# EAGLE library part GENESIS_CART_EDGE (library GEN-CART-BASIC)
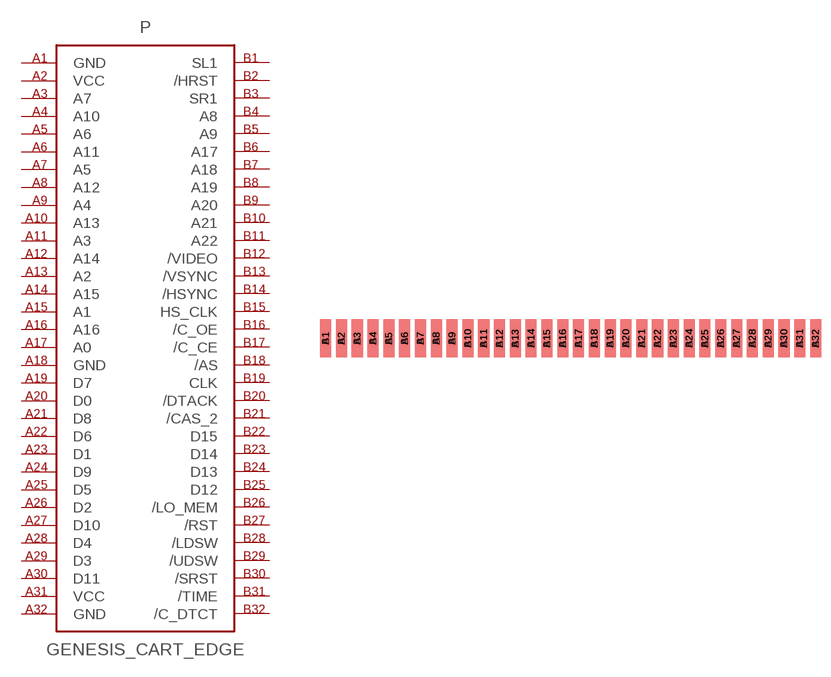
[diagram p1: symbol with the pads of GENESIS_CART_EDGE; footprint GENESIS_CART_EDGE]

Designator prefix P

## GENESIS_CART_EDGE  [GENESIS_CART_EDGE]
A1  GND  pwr
A2  VCC  pwr
A3  A7  in
A4  A10  in
A5  A6  in
A6  A11  in
A7  A5  in
A8  A12  in
A9  A4  in
A10  A13  in
A11  A3  in
A12  A14  in
A13  A2  in
A14  A15  in
A15  A1  in
A16  A16  in
A17  A0  in
A18  GND  pwr
A19  D7
A20  D0
A21  D8
A22  D6
A23  D1
A24  D9
A25  D5
A26  D2
A27  D10
A28  D4
A29  D3
A30  D11
A31  VCC  pwr
A32  GND  pwr
B1  SL1  in
B2  /HRST  out
B3  SR1  in
B4  A8  in
B5  A9  in
B6  A17  in
B7  A18  in
B8  A19  in
B9  A20  in
B10  A21  in
B11  A22  in
B12  /VIDEO  in
B13  /VSYNC  in
B14  /HSYNC  in
B15  HS_CLK  in
B16  /C_OE  in
B17  /C_CE  in
B18  /AS  in
B19  CLK  in
B20  /DTACK  out
B21  /CAS_2  in
B22  D15
B23  D14
B24  D13
B25  D12
B26  /LO_MEM  in
B27  /RST  in
B28  /LDSW  in
B29  /UDSW  in
B30  /SRST  out
B31  /TIME  in
B32  /C_DTCT  out

## Footprint GENESIS_CART_EDGE (pad centres in mm)
smd 1.778 x 6.096 bottom: A1 -38.1,0; A2 -35.56,0; A3 -33.02,0; A4 -30.48,0; A5 -27.94,0; A6 -25.4,0; A7 -22.86,0; A8 -20.32,0; A9 -17.78,0; A10 -15.24,0; A11 -12.7,0; A12 -10.16,0; A13 -7.62,0; A14 -5.08,0; A15 -2.54,0; A16 0,0; A17 2.54,0; A18 5.08,0; A19 7.62,0; A20 10.16,0; A21 12.7,0; A22 15.24,0; A23 17.78,0; A24 20.32,0; A25 22.86,0; A26 25.4,0; A27 27.94,0; A28 30.48,0; A29 33.02,0; A30 35.56,0; A31 38.1,0; A32 40.64,0
smd 1.778 x 6.096: B1 -38.1,0; B2 -35.56,0; B3 -33.02,0; B4 -30.48,0; B5 -27.94,0; B6 -25.4,0; B7 -22.86,0; B8 -20.32,0; B9 -17.78,0; B10 -15.24,0; B11 -12.7,0; B12 -10.16,0; B13 -7.62,0; B14 -5.08,0; B15 -2.54,0; B16 0,0; B17 2.54,0; B18 5.08,0; B19 7.62,0; B20 10.16,0; B21 12.7,0; B22 15.24,0; B23 17.78,0; B24 20.32,0; B25 22.86,0; B26 25.4,0; B27 27.94,0; B28 30.48,0; B29 33.02,0; B30 35.56,0; B31 38.1,0; B32 40.64,0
